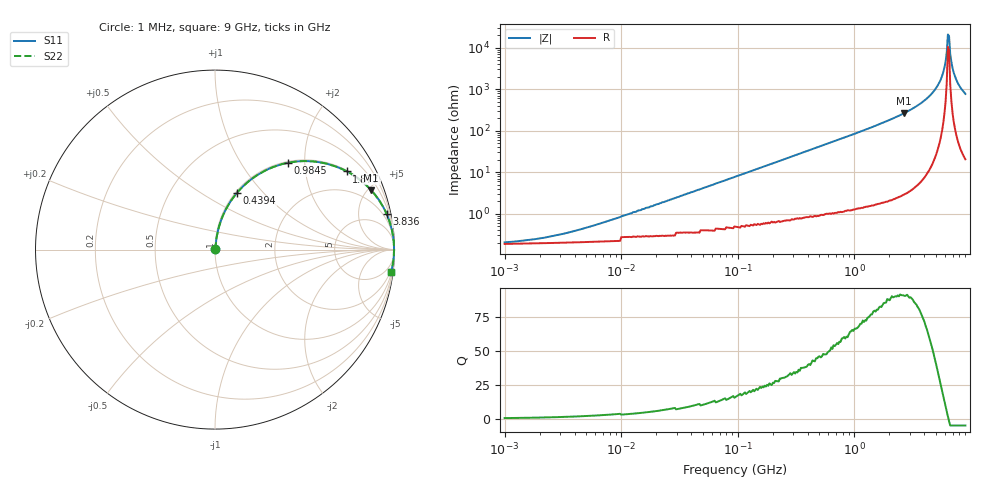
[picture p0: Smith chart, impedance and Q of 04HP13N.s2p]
# MHz S MA R 50
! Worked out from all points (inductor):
!   396 points, 1 MHz to 9 GHz, reference 50 ohm
!   read as one part in series: L = 13 nH near 8.147 MHz
!   highest Q = 91.3 at 2.653 GHz (marker M1), where L = 15.6 nH
!   self-resonance near 6.369 GHz
!   S11 on the Smith chart (normalised r, x): 1 MHz: 1.00, +0.00; 439.4 MHz: 1.02, +0.72; 984.5 MHz: 1.03, +1.65; 1.877 GHz: 1.04, +3.35; 3.836 GHz: 1.12, +9.71; 9 GHz: 1, -15
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1  0.001919 25.1  0.998 -0.0  0.998 -0.0  0.001919 25.1
2.14  0.002575 42.5  0.998 -0.1  0.998 -0.1  0.002575 42.5
4.578  0.004293 60.2  0.998 -0.2  0.998 -0.2  0.004293 60.2
20.961  0.017 79.2  0.997 -1.0  0.997 -1.0  0.017 79.2
95.968  0.078 82.1  0.992 -4.5  0.992 -4.5  0.078 82.1
439.375  0.337 69.0  0.934 -19.7  0.934 -19.7  0.337 69.0
984.49  0.631 50.0  0.766 -39.1  0.766 -39.1  0.631 50.0
1877.207  0.854 30.6  0.51 -58.7  0.51 -58.7  0.854 30.6
2011.613  0.872 28.6  0.479 -60.7  0.479 -60.7  0.872 28.6
2652.609  0.93 20.9  0.357 -68.5  0.357 -68.5  0.93 20.9
3835.704  0.977 11.6  0.201 -77.6  0.201 -77.6  0.977 11.6
4830.06  0.992 6.3  0.11 -82.5  0.11 -82.5  0.992 6.3
5546.474  0.996 3.3  0.057 -84.4  0.057 -84.4  0.996 3.3
6082.189  0.997 1.2  0.022 -82.5  0.022 -82.5  0.997 1.2
6224.015  0.998 0.7  0.013 -78.8  0.013 -78.8  0.998 0.7
6369.149  0.998 0.2  0.00478 -59.5  0.00478 -59.5  0.998 0.2
6517.667  0.998 -0.3  0.005224 61.8  0.005224 61.8  0.998 -0.3
6669.648  0.997 -0.8  0.014 78.7  0.014 78.7  0.997 -0.8
6825.172  0.997 -1.3  0.022 82.2  0.022 82.2  0.997 -1.3
7147.186  0.997 -2.3  0.04 83.9  0.04 83.9  0.997 -2.3
7837.509  0.994 -4.3  0.075 83.5  0.075 83.5  0.994 -4.3
9000  0.988 -7.4  0.128 81.1  0.128 81.1  0.988 -7.4
